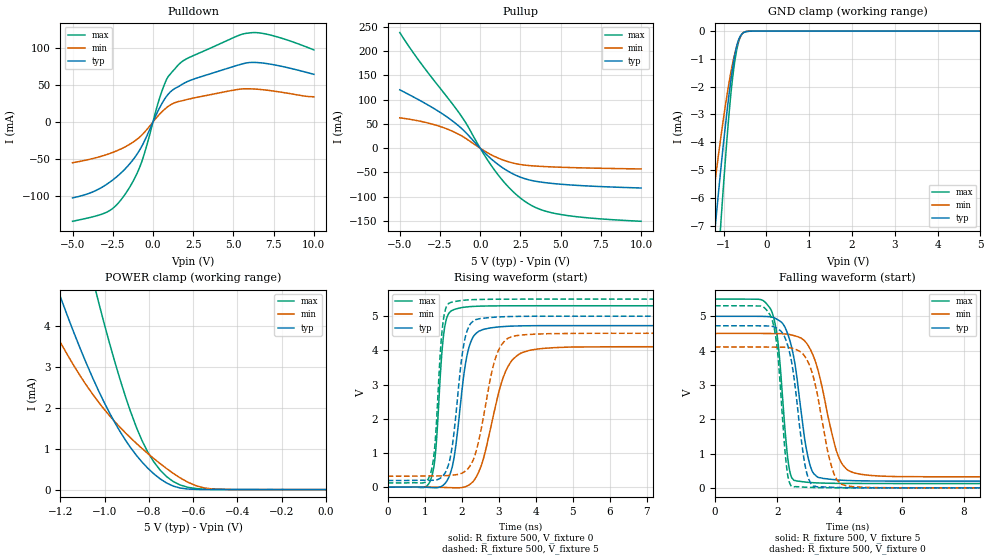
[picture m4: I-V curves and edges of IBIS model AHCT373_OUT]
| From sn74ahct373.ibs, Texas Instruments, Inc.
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[Model]   AHCT373_OUT
Model_type  3-state
Enable   Active-Low
Vref =   0
Rref =   1000
Cref =   50p
Vmeas =   1.5
| variable   typ   min   max
C_comp   2.26pF   2.03pF   2.35pF
| C_pullup   3.56pF   2.17pF   4.82pF
| C_pulldown   3.93pF   2.38pF   6.45pF
| C_tri-state   2.26pF   2.03pF   2.35pF
[Temperature Range]   40   100   -40
| Ambient temperature   25   85   -40
[Voltage range]   5   4.5   5.5
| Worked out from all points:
|   slope of the pulldown table from 0 to 0.75 V, typ, clamps not added: 23.6 ohm
|   slope of the pullup table from 0 to 0.75 V, typ, clamps not added: 31.3 ohm
|   GND clamp passes 1 mA (typ) near -0.75 V on its own axis
|   POWER clamp passes 1 mA (typ) near -0.88 V on its own axis
|   rising waveform, R_fixture 500, V_fixture 0: 20-80 % time 325ps typ, 566ps min, 194ps max; typ from 0 V to 4.72 V
|   falling waveform, R_fixture 500, V_fixture 5: 20-80 % time 453ps typ, 643ps min, 299ps max; typ from 5 V to 0.196 V
|   rising waveform, R_fixture 500, V_fixture 5: 20-80 % time 298ps typ, 467ps min, 184ps max; typ from 0.196 V to 5 V
|   falling waveform, R_fixture 500, V_fixture 0: 20-80 % time 405ps typ, 542ps min, 275ps max; typ from 4.72 V to 0 V
[GND Clamp]
| AHCT373_OUT
|   Voltage   I(typ)   I(min)   I(max)
-5V       -97.16mA   -69.47mA   -118.1mA
-1.335V   -9.481mA   -7.134mA   -13.38mA
-1.31V    -9.038mA   -6.811mA   -12.76mA
-1.205V   -7.232mA   -5.494mA   -10.21mA
-1.175V   -6.734mA   -5.129mA   -9.491mA
-1.075V   -5.137mA   -3.955mA   -7.178mA
-1.055V   -4.831mA   -3.729mA   -6.73mA
-870mV    -2.26mA    -1.837mA   -2.948mA
-765mV    -1.108mA   -993.9uA   -1.396mA
-650mV    -318.6uA   -348.4uA   -399.3uA
-510mV    -37.58uA   -31.6uA    -34.57uA
5V        31.12nA    10.43uA    284.5nA
[POWER Clamp]
| AHCT373_OUT
|   Voltage   I(typ)   I(min)   I(max)
-5V       119mA      83.04mA    180mA
-1.315V   6.531mA    4.817mA    11.72mA
-1.195V   4.641mA    3.553mA    8.506mA
-1.055V   2.743mA    2.339mA    5.178mA
-1.03V    2.446mA    2.156mA    4.639mA
-930mV    1.416mA    1.521mA    2.687mA
-855mV    827.5uA    1.123mA    1.501mA
-780mV    396.3uA    769.7uA    694.8uA
-720mV    161.3uA    514.3uA    317uA
-625mV    14.65uA    183.5uA    57.66uA
-515mV    819.5nA    16.06uA    5.129uA
-84.45fV  31.12nA    1.807nA    433.1nA
[Pulldown]
| AHCT373_OUT
|   Voltage   I(typ)   I(min)   I(max)
-5V       -102.3mA   -54.86mA   -133.8mA
-2.815V   -83.04mA   -43.41mA   -120.8mA
-1.71V    -62.74mA   -33.25mA   -96.72mA
-1.15V    -48.25mA   -25.84mA   -76.29mA
-715mV    -33.55mA   -18.08mA   -54.64mA
310mV     14.74mA    8.08mA     24.97mA
780mV     32.72mA    18.17mA    54.14mA
1.835V    51.04mA    28.7mA     81.78mA
5.265V    76.49mA    43.83mA    116.1mA
6.135V    80.3mA     44.65mA    120.3mA
7.58V     76.86mA    41.45mA    115.6mA
10V       64.23mA    34mA       97.15mA
[Pullup]
| AHCT373_OUT
|   Voltage   I(typ)   I(min)   I(max)
-5V       120.4mA    62.69mA    238.5mA
-3.72V    97.96mA    55.59mA    176.6mA
-1.735V   56.47mA    35.11mA    91.68mA
-930mV    33.48mA    20.83mA    54.07mA
125mV     -4.363mA   -2.727mA   -6.908mA
890mV     -27.85mA   -16.92mA   -45.14mA
1.71V     -47mA      -27.58mA   -78.37mA
2.525V    -60.03mA   -33.77mA   -103.5mA
3.535V    -68.63mA   -36.97mA   -123.6mA
4.77V     -73.58mA   -38.95mA   -135.3mA
6.78V     -77.99mA   -40.87mA   -143.8mA
10V       -82.05mA   -42.74mA   -150.7mA
[Ramp]
| AHCT373_OUT
| variable   typ   min   max
dV/dt_r   2.85/3.29E-10   2.48/5.80E-10   3.19/1.99E-10
dV/dt_f   2.88/4.67E-10   2.51/6.46E-10   3.22/3.01E-10
R_load = 500
[Rising Waveform]
| AHCT373_OUT
R_fixture =   500
C_fixture =   0
L_fixture =   0
V_fixture =   0
V_fixture_min = 0
V_fixture_max = 0
|   Time   V(typ)   V(min)   V(max)
0s        -36.17uV   -47.34uV   -18.92uV
1.155ns   -9.873mV   5.753mV    197mV
1.29ns    -17.64mV   1.402mV    978.6mV
1.565ns   127.9mV    -8.826mV   4.817V
1.8ns     902.2mV    -17.25mV   5.197V
2.125ns   3.745V     25.33mV    5.271V
2.525ns   4.588V     612.9mV    5.296V
3.25ns    4.706V     3.525V     5.306V
4.195ns   4.725V     4.058V     5.307V
50ns      4.724V     4.106V     5.306V
[Falling Waveform]
| AHCT373_OUT
R_fixture =   500
C_fixture =   0
L_fixture =   0
V_fixture =   5
V_fixture_min = 4.5
V_fixture_max = 5.5
|   Time   V(typ)   V(min)   V(max)
0s        5V         4.5V       5.5V
1.8ns     4.982V     4.497V     5.191V
2.02ns    4.898V     4.494V     4.277V
2.395ns   4.327V     4.468V     523.8mV
2.585ns   3.525V     4.425V     211.9mV
2.865ns   1.534V     4.296V     172.1mV
3.175ns   411.7mV    3.809V     148.7mV
4.02ns    225.6mV    805.3mV    129.6mV
4.965ns   200.6mV    363.8mV    126.3mV
50ns      196.2mV    321.4mV    126mV
[Rising Waveform]
| AHCT373_OUT
R_fixture =   500
C_fixture =   0
L_fixture =   0
V_fixture =   5
V_fixture_min = 4.5
V_fixture_max = 5.5
|   Time   V(typ)   V(min)   V(max)
0s        196.2mV    321.4mV    126mV
1.155ns   200.5mV    329.1mV    389.5mV
1.265ns   205.9mV    328.9mV    1.094V
1.555ns   422mV      336.2mV    5.173V
1.75ns    1.231V     352.1mV    5.415V
2.055ns   4.157V     438.2mV    5.468V
2.385ns   4.904V     1.028V     5.488V
2.99ns    4.978V     3.989V     5.498V
3.675ns   4.998V     4.457V     5.5V
50ns      5V         4.5V       5.5V
[Falling Waveform]
| AHCT373_OUT
R_fixture =   500
C_fixture =   0
L_fixture =   0
V_fixture =   0
V_fixture_min = 0
V_fixture_max = 0
|   Time   V(typ)   V(min)   V(max)
0s        4.724V     4.106V     5.306V
1.8ns     4.712V     4.102V     4.987V
2.005ns   4.642V     4.1V       4.03V
2.32ns    4.199V     4.093V     471mV
2.54ns    3.201V     4.05V      30.22mV
2.875ns   745.6mV    3.848V     19.81mV
3.07ns    145.4mV    3.494V     11.67mV
3.815ns   14.15mV    431.3mV    1.671mV
4.455ns   2.742mV    33.47mV    152uV
50ns      -36.68uV   -48.19uV   -19.04uV
